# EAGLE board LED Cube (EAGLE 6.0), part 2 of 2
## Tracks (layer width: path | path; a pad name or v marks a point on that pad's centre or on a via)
GND  (via drill 0.4)
  Top 0.406: IC6.1 146.54,70.66 v146.7,70.5 | IC5.1 146.21,53.59 v146.5,53.3 | IC3.1 145.82,35.08 v146.3,34.6 | v146.3,17.6 145.78,18.11 IC2.1 143.08,16.45 140.45,16.45 | C5.1 25.29,76.88 C4.1 25.76,76.86 v26.7,77.8 | C6.1 19.52,72.69 C7.1 | C7.1 19.74,70.77 C9.1 | C7.1 19.74,73.74 C8.1 | C8.1 19.88,74.99 R10.2 17.82,76.88 IC10.18 11.72,76.88 11.4,77.2 11.4,78.7 | C8.1 21.79,74.99 v22,75.2 | X2.5 10.34,92.66 11,92 11,82.6 11.45,82.15 | 11.45,82.15 11.5,82.1 | 11.5,82.1 13.09,82.1 IC10.26 | IC10.25 12.18,81.42 11.5,82.1 | 11.4,78.7 11.4,79.4 | 11.4,79.4 11.4,82.1 11.45,82.15 | IC10.21 11.53,78.83 11.4,78.7 | IC10.7 11.32,79.47 11.4,79.4 | IC11.PC IC11.PB | IC11.PD IC11.PC | IC11.PC 50.73,59.02 v50.9,59.2 50.45,58.75 C22.1 | v43.9,78.1 43.84,78.16 IC14.6 41.46,78.2 35.5,78.2 35.03,78.67 C1.1 | IC14.39 47.3,81.8 v47.2,81.7 | v51,78.3 51.14,78.16 IC14.28 53.16,78.1 60.7,78.1 | IC14.18 v48.1,74.5 | 60.7,78.1 60.9,78.1 62.02,76.98 C2.2 63.1,76.44 U$74.B2 U$74.B | C3.2 60.14,77.54 60.7,78.1 | R27.2 18.99,39.51 v19.3,39.2 | R28.2 27.19,39.51 v27.3,39.4 | R29.2 35.39,39.51 v35.6,39.3 | R30.2 43.49,39.51 v43.7,39.3 | v19.7,52.9 19.59,53.01 R23.2 18.28,50.82 U$70.3 | R24.2 27.29,52.91 v27.4,52.8 | R25.2 v35.89,52.81 v35.9,52.8 | R26.2 43.69,52.71 v43.9,52.5 | C14.2 34.91,21.12 C15.2 35.52,22.48 v36.3,21.7 | R31.1 53.49,11.37 R21.1 53.03,11.33 v52,10.3 | C12.2 26.14,16.24 24.15,14.25 | 24.15,14.25 24.1,14.2 24.1,11.7 23.1,10.7 20.17,10.7 IC12.2 | C10.1 21.86,16.54 24.15,14.25 | C11.2 34.61,8.11 v35,8.5 | 44.3,25.19 IC1.3 51.8,25.2 52.61,24.39 IC1.21 57.64,24.39 C18.2 59.64,24.74 C17.2 60.49,23.91 59.7,24.7 57.8,24.7 57.8,24.5 57.7,24.4 54.3,24.4 v53.6,23.7
  Top 0.406: 44.3,25.19 43.84,25.19 C16.2 | IC1.5 45.9,23.59 44.3,25.19 | C19.2 5.4,31.55 C20.2 3.85,32.7 IC13.GND | R14.1 47.7,67.2 v47.9,67.4 | IC9.10 77.13,84.27 78.5,82.9 C23.1 80.65,83.95 v80.1,84.5 | IC9.1 79.42,96.97 v79.7,96.7 | IC8.10 79.14,65.1 C24.1 80.35,66.15 v79.8,66.7 | IC8.1 79.14,78.83 v79.5,79.2 | IC4.10 76.45,44.85 77.2,44.1 80.25,44.1 C25.1 80.35,45.15 v80,45.5 | IC4.1 78.67,58.27 v79.4,59 | C26.1 78.3,22.7 78.2,22.8 | 76.5,24.5 76.5,25.2 IC7.10 76.55,24.55 76.5,24.5 | IC7.1 78.69,36.69 v79.1,37.1 | 76.5,24.5 78.2,22.8 | 78.2,22.8 78.2,23.6 v78.4,23.8 | C27.1 140.45,16.45 | 140.45,16.45 139,17.9 139,29 139.6,29.6 144.69,29.6 IC2.10 | v142,32.6 C28.1 140.5,32.65 140.5,34.7 138.7,36.5 138.7,45.7 139.5,46.51 IC3.10 | v142.2,50.9 142.1,51 C29.1 140.6,51.05 140.6,53.3 138.8,55.1 138.8,64.3 139.53,65.03 IC5.10 | v142.5,68.4 142.3,68.2 C30.1 140.7,68.25 140.7,81.3 141.49,82.08 IC6.10
  Bottom 0.406: v146.7,70.5 146.5,70.5 | v146.5,53.3 146.1,53.3 | v146.3,34.6 146,34.6 | v146.3,17.6 145.9,17.6 | v26.7,77.8 26.2,77.8 | v22,75.2 21.9,75.2 21.8,75.3 | v50.9,59.2 53.5,59.2 | v43.9,78.1 43.6,78.1 | v47.2,81.7 47.2,82.1 47.3,82.2 | v51,78.3 51.3,78.3 51.4,78.2 | v48.1,74.5 48.1,74 48.2,74 | v19.3,39.2 18.9,39.2 18.8,39.1 | v27.3,39.4 27.1,39.4 26.9,39.2 | v35.6,39.3 35.5,39.3 35.3,39.1 | v43.7,39.3 43.6,39.3 43.3,39 | v19.7,52.9 19.5,52.9 19.4,52.8 | v27.4,52.8 27.2,52.8 27.1,52.7 | v35.9,52.8 35.9,52.7 35.7,52.5 | v43.9,52.5 43.8,52.5 43.7,52.4 | v36.3,21.7 35.7,21.7 | v52,10.3 52,10.8 | v35,8.5 34.6,8.5 | v47.9,67.4 47.9,67 48,66.9 | v80.1,84.5 80.1,84 | v79.7,96.7 79.3,96.7 79.2,96.6 | v79.8,66.7 79.8,66.1 | v79.5,79.2 79.2,79.2 79.1,79.3 | v80,45.5 80,45.2 | v79.4,59 78.6,59 | v79.1,37.1 78.7,37.1 78.6,37.2 | v78.4,23.8 78.4,23.5 | v142,32.6 142,32.2 | v142.2,50.9 142,50.9 | v142.5,68.4 142.1,68.4 | v53.6,23.7 53.6,24
  pour Bottom (isolate 0.4): 0,0 160,0 160,100 0,100
  pour Top (isolate 0.4): 0,0 160,0 160,100 0,100
N$1  (via drill 0.4)
  Top 0.406: U$3.P$3 99.96,32.54 100.8,31.7 104.9,31.7 108.2,28.4 108.2,22.2 108.4,22 108.4,21.1 107.1,19.8 v107.1,19.5
  Bottom 0.406: v107.1,19.5 111.09,19.5 SV1.4
N$2
  Top 0.406: IC14.4 36.94,79.76 32.5,84.2 32.5,86.2 | 32.5,86.2 32.5,93.72 JP3.5 | R1.2 32.5,86.2
N$3
  Top 0.406: IC14.29 62.28,78.96 C2.1
N$4  (via drill 0.4)
  Top 0.406: IC6.2 150.07,71.92 150.5,71.5 v150.5,55 v150.5,36.3 v150.5,19.4 150.5,10.8 149.7,10 106.3,10 104.5,11.8 104.5,14.8 99.3,20 75.7,20 72.4,23.3 72.4,25.3 74,25.3 74.2,25.5 74.2,25.6 74.4,25.8 v74.4,36 v74.4,57.1 v74.4,77.8 74.4,95.4 74.5,95.5 | v142.2,55 144.81,55 IC5.2 | IC2.2 140.81,19.39 v140.8,19.4 | IC7.2 80.58,35.41 v80.6,35.4 | IC4.2 v80.39,56.99 v80.4,57 | IC8.2 80.86,77.56 v80.9,77.6 | 74.5,95.5 74.7,95.7 IC9.2 | IC14.37 48.9,87.1 51.6,89.8 57.5,89.8 57.9,90.2 57.9,92 61.5,95.6 74.4,95.6 74.5,95.5 | IC3.2 142.06,36.34 v142,36.4
  Bottom 0.406: v150.5,55 v142.2,55 | v140.8,19.4 v150.5,19.4 | v80.6,35.4 75,35.4 v74.4,36 | v80.4,57 74.5,57 v74.4,57.1 | v80.9,77.6 74.6,77.6 v74.4,77.8 | v142,36.4 150.4,36.4 v150.5,36.3
N$5  (via drill 0.4)
  Top 0.406: IC6.3 151.1,73.19 151.5,72.8 v151.5,56.2 v151.5,37.6 v151.5,20.6 151.5,10.7 150.1,9.3 105.8,9.3 103.6,11.5 103.6,14.5 99,19.1 75.4,19.1 71.7,22.8 71.7,25.5 72.2,26 73.1,26 73.4,26.3 v73.4,34.8 v73.4,55.9 v73.4,76.6 v73.4,94.5 61.6,94.5 58.8,91.7 58.8,89.4 58.3,88.9 52,88.9 49.7,86.6 IC14.36 | v140.9,56.2 144.88,56.2 IC5.3 | IC2.3 142.16,20.66 v142.1,20.6 | IC7.3 79.25,34.15 v79.3,34.2 | IC4.3 79.12,55.73 v79.2,55.8 | IC8.3 v79.69,76.3 v79.7,76.3 | v81.2,94.5 77.2,94.5 IC9.3 | IC3.3 140.72,37.62 v140.7,37.6
  Bottom 0.406: v151.5,56.2 v140.9,56.2 | v142.1,20.6 v151.5,20.6 | v79.3,34.2 74,34.2 v73.4,34.8 | v79.2,55.8 73.5,55.8 v73.4,55.9 | v79.7,76.3 73.7,76.3 v73.4,76.6 | v73.4,94.5 v81.2,94.5 | v140.7,37.6 v151.5,37.6
N$6  (via drill 0.4)
  Top 0.406: IC6.4 152.13,74.47 152.3,74.3 v152.3,57.4 v152.3,38.9 v152.3,21.9 152.3,10.3 150.7,8.7 146.3,8.6 105.4,8.6 102.8,11.2 102.8,14.2 98.6,18.4 75,18.4 71,22.4 71,25.9 71.8,26.7 72.2,26.7 72.4,26.9 v72.4,32.6 v72.4,54.3 v72.4,75.1 v72.4,93.2 61.7,93.2 59.7,91.2 59.7,88.8 58.9,88 52.3,88 50.5,86.2 IC14.35 | v142.2,57.4 IC5.4 | IC3.4 141.91,38.88 v141.9,38.9 | IC7.4 80.47,32.88 v80.5,32.9 | IC4.4 80.34,54.45 v80.4,54.4 | IC8.4 80.78,75.03 v80.8,75 | v79.8,93.2 77.17,93.2 IC9.4 | IC2.4 140.88,21.93 v140.8,22
  Bottom 0.406: v152.3,57.4 v142.2,57.4 | v141.9,38.9 v152.3,38.9 | 152.1,21.9 152.2,22 | 152.28,21.93 v152.3,21.9 152.2,22 | v80.5,32.9 72.7,32.9 v72.4,32.6 | v80.4,54.4 72.5,54.4 v72.4,54.3 | v80.8,75 72.5,75 v72.4,75.1 | v72.4,93.2 v79.8,93.2 | v140.8,22 152.2,22
N$7
  Top 0.406: IC14.7 32.63,77.36 Q1.2 25.41,79.94 C5.2
N$8
  Top 0.406: IC14.8 31.49,76.56 Q1.1 25.35,75.12 C4.2
N$9  (via drill 0.4)
  Top 0.406: IC6.5 152.97,75.73 153.2,75.5 153.2,58.8 v153.1,58.7 | v140.9,58.7 144.92,58.7 IC5.5 | IC3.5 140.84,40.16 v140.8,40.2 | v153.1,58.7 v153.1,40.2 v153.1,23.2 | IC2.5 v142.1,23.2 | v153.1,58.7 153.1,9.9 151.2,8 104.9,8 102,10.9 102,13.9 98.2,17.7 74.6,17.7 70.3,22 70.3,26.1 71.1,26.9 v71.1,32.1 v71.1,53.4 v71.1,73.8 71.1,91.8 | IC7.5 79.11,31.61 v79.2,31.7 | IC4.5 78.89,53.19 v79,53.3 | IC8.5 79.56,73.75 v79.6,73.8 | 71.1,91.8 v71.2,91.9 | v81,91.9 IC9.5 | 71.1,91.8 62.3,91.8 60.7,90.2 60.7,88.2 59.6,87.1 52.8,87.1 51.3,85.6 IC14.34
  Bottom 0.406: v140.8,40.2 v153.1,40.2 | v142.1,23.2 v153.1,23.2 | v79.2,31.7 71.5,31.7 v71.1,32.1 | v79,53.3 71.2,53.3 v71.1,53.4 | v79.6,73.8 v71.1,73.8 | v71.2,91.9 v81,91.9 | v153.1,58.7 144.97,58.7 IC5.5 140.93,58.67 v140.9,58.7 v153.1,58.7
N$10  (via drill 0.4)
  Top 0.406: IC6.6 153.79,77 154,76.8 v154,60 v154,41.6 v154,24.6 154,9.5 151.7,7.2 104.5,7.2 101.1,10.6 101.1,13.5 97.8,16.8 74.2,16.8 69.4,21.6 69.4,26.8 69.5,26.9 69.6,26.9 69.7,27 v69.7,30.4 v69.7,52.2 v69.7,72.9 v69.7,90.6 69.6,90.7 62.6,90.7 61.8,89.9 61.8,83 60.96,82.16 IC14.33 | v142.2,60 144.89,60 IC5.6 | IC3.6 142.07,41.42 v142,41.5 | IC2.6 140.94,24.46 v140.8,24.6 | IC7.6 80.33,30.34 v80.4,30.4 | IC4.6 80.28,51.91 v80.3,51.9 | IC8.6 80.78,72.48 v80.8,72.5 | v79.7,90.6 77.16,90.6 IC9.6
  Bottom 0.406: v154,60 v142.2,60 | v142,41.5 154,41.5 v154,41.6 | v140.8,24.6 v154,24.6 | v80.4,30.4 v69.7,30.4 | v80.3,51.9 70,51.9 v69.7,52.2 | v80.8,72.5 70.1,72.5 v69.7,72.9 | v69.7,90.6 v79.7,90.6
N$11  (via drill 0.4)
  Top 0.406: IC6.7 154.62,78.28 154.8,78.1 v154.8,61.2 v154.8,42.7 v154.8,25.8 154.8,9.1 152.2,6.5 152.2,6.4 104.1,6.4 100.2,10.3 100.2,13.2 97.4,16 73.7,16 68.5,21.2 68.5,26.9 68.2,27.2 v68.2,28.9 v68.2,51 v68.2,71.2 v68.2,89.4 63.4,89.4 62.6,88.6 62.6,82.5 61.46,81.36 IC14.32 | v140.9,61.2 144.93,61.2 IC5.7 | IC2.7 142.16,25.73 v142.1,25.8 | IC7.7 78.97,29.07 v79,29.1 | IC4.7 78.94,50.65 v79,50.7 | IC8.7 79.39,71.22 v79.4,71.2 | v81.1,89.4 77.18,89.4 IC9.7 | IC3.7 v140.71,42.7 v140.7,42.7
  Bottom 0.406: v154.8,61.2 v140.9,61.2 | v142.1,25.8 v154.8,25.8 | v79,29.1 68.4,29.1 v68.2,28.9 | v79,50.7 68.5,50.7 v68.2,51 | v79.4,71.2 v68.2,71.2 | v68.2,89.4 v81.1,89.4 | v154.79,42.7 v154.8,42.7 v140.7,42.7
N$12  (via drill 0.4)
  Top 0.406: IC6.8 155.35,79.55 155.6,79.3 v155.6,62.5 v155.6,44.1 v155.6,26.9 155.6,8.5 152.7,5.6 103.6,5.6 99.1,10.1 99.1,13 96.9,15.2 73.2,15.2 67.4,21 67.4,26.5 66.6,27.3 v66.6,27.8 v66.6,49.3 v66.6,69.7 v66.6,88.2 64.3,88.2 63.5,87.4 63.5,82.1 61.96,80.56 IC14.31 | v142.2,62.5 144.93,62.5 IC5.8 | IC3.8 142.13,43.97 v142.1,44 | IC7.8 v80.39,27.8 v80.4,27.8 | IC4.8 80.28,49.38 v80.3,49.4 | IC8.8 80.56,69.94 v80.6,69.9 | v79.8,88.1 77.15,88.1 IC9.8 | IC2.8 v140.5,27
  Bottom 0.406: v155.6,62.5 v142.2,62.5 | v142.1,44 155.5,44 v155.6,44.1 | v80.4,27.8 v66.6,27.8 | v80.6,69.9 66.8,69.9 v66.6,69.7 | v66.6,88.2 79.7,88.2 v79.8,88.1 | v140.5,27 155.6,27 v155.6,26.9 | v80.3,49.4 66.6,49.4 v66.6,49.3
N$13  (via drill 0.4)
  Top 0.406: IC6.9 155.69,80.81 156.4,80.1 v156.4,63.7 | v140.9,63.8 144.9,63.8 IC5.9 | IC3.9 140.76,45.23 v140.7,45.3 | v156.4,63.7 v156.4,45.5 v156.4,28.4 | IC2.9 142.03,28.27 v142,28.3 | v156.4,63.7 156.4,8 153.3,4.9 103.3,4.9 98.4,9.8 98.4,12.6 96.5,14.5 72.7,14.5 66.5,20.7 66.5,25.6 64.9,27.2 v64.9,27.3 v64.9,48.1 v64.9,68.8 64.9,79.8 | IC7.9 78.83,26.52 v78.9,26.6 | IC4.9 v78.89,48.1 v78.9,48.1 | IC8.9 79.28,68.67 v79.3,68.7 | 64.9,79.8 64.9,86.7 v65,86.8 | v81,86.9 77.22,86.9 IC9.9 | IC14.30 64.86,79.76 64.9,79.8
  Bottom 0.406: v140.7,45.3 156.2,45.3 v156.4,45.5 | v142,28.3 156.3,28.3 v156.4,28.4 | v78.9,26.6 65.6,26.6 v64.9,27.3 | v78.9,48.1 v64.9,48.1 | v79.3,68.7 65,68.7 v64.9,68.8 | v65,86.8 80.9,86.8 v81,86.9 | v156.4,63.7 141,63.7 v140.9,63.8 156.3,63.8 v156.4,63.7
N$14  (via drill 0.4)
  Top 0.406: IC9.11 87.19,84.99 v86.3,84.1 | v59.1,85.1 54.3,85.1 v52.7,83.5 | v44.9,87.7 45.3,87.7 45.7,87.3 IC14.41
  Bottom 0.406: v86.3,84.1 86.3,83.6 85.4,82.7 61.5,82.7 v59.1,85.1 | v52.7,83.5 49.1,83.5 v44.9,87.7
N$15  (via drill 0.4)
  Top 0.406: IC8.11 86.89,65.59 v86,64.7 | v44.9,81.7 IC14.42 | v57.3,59.6 61.7,59.6 v62.3,59
  Bottom 0.406: v44.9,81.7 45.1,81.5 45.1,66.4 46.8,64.7 55.3,64.7 57.5,62.5 57.5,59.8 v57.3,59.6 | v62.3,59 63.1,59 68.65,64.55 68.8,64.7 v86,64.7
N$16  (via drill 0.4)
  Top 0.406: IC6.11 134.99,83.11 v132.8,85.3 | IC14.21 50.5,74.2 v49.3,75.4 | v46.2,77.3 46.2,77.2 v43.4,74.4 | v71,11.2 82.5,11.2 v84.8,8.9
  Bottom 0.406: v132.8,85.3 130.6,85.3 125.3,80 125.3,11.7 122.4,8.8 97,8.8 96.9,8.9 v84.8,8.9 | v49.3,75.4 49.3,77.6 48.4,78.5 47.4,78.5 v46.2,77.3 | v43.4,74.4 43.4,65.5 44.1,64.8 44.1,57.5 46.5,55.1 48.1,55.1 53.3,49.9 53.3,47.7 59.2,41.8 59.2,24.3 61.5,22 64.9,22 70.6,16.3 70.6,11.6 v71,11.2
N$17  (via drill 0.4)
  Top 0.406: IC5.11 134.18,65.03 v132.6,66.6 | IC14.22 53.16,72.36 v53.6,72.8 | v54,83.1 v58.8,83.1 | v63.2,48.5 63.2,26.8 v64.6,25.4
  Bottom 0.406: v132.6,66.6 127.5,66.6 126.5,65.6 126.5,11.3 122.7,7.5 83.7,7.5 65.8,25.4 v64.6,25.4 | v53.6,72.8 53.6,82.7 v54,83.1 | v58.8,83.1 58.8,82.2 63.4,77.6 63.4,66.4 61.4,64.4 61.4,58.5 63.4,56.5 63.4,48.7 v63.2,48.5
N$18  (via drill 0.4)
  Top 0.406: IC4.11 86.51,44.71 v85.4,43.6 | v60.3,62.8 60.3,66.7 v60.4,66.8 | v57.4,74.1 53.16,74.1 IC14.23
  Bottom 0.406: v85.4,43.6 65.3,43.6 60.3,48.6 v60.3,62.8 | v60.4,66.8 60.4,71.1 v57.4,74.1
N$19  (via drill 0.4)
  Top 0.406: IC3.11 133.59,46.51 v132.5,47.6 | IC14.24 50.94,74.96 v50.6,75.3 | v46.4,79.9 v43,79.9 | v74,6.3 v80.5,6.3
  Bottom 0.406: v132.5,47.6 128.7,47.6 127.9,46.8 127.9,11 123.2,6.3 v80.5,6.3 | v50.6,75.3 50.6,77.4 48.2,79.8 46.5,79.8 v46.4,79.9 | v43,79.9 43,79.1 41.6,77.6 41.6,66.2 43.3,64.5 43.3,57.1 46,54.4 47.7,54.4 52.5,49.6 52.5,47.3 58.4,41.4 58.4,23.9 61.2,21.1 64.6,21.1 69.8,15.9 69.8,10.5 v74,6.3
N$20  (via drill 0.4)
  Top 0.406: IC2.11 134.16,29.55 v133.1,30.6 | v53.9,62.7 53.8,62.7 53.3,63.2 53.3,66.7 v53.1,66.9 | v48.3,76.6 50.4,76.6 51.2,75.8 53.06,75.8 IC14.25
  Bottom 0.406: v133.1,30.6 130.7,30.6 129.3,29.2 129.3,10.6 123.8,5.1 79.1,5.1 71.5,12.7 71.5,16.6 60.2,27.9 60.2,42.1 54.6,47.7 54.6,62 v53.9,62.7 | v53.1,66.9 53.1,66.6 52.1,65.6 47.3,65.6 46,66.9 46,74.3 v48.3,76.6
N$21  (via drill 0.4)
  Top 0.406: IC7.11 86.61,24.39 v87.8,23.2 | v58.5,67.3 58.7,67.3 61.2,69.8 61.2,74.4 v60.5,75.1 | v56.9,76.4 56.8,76.4 56.6,76.6 53.14,76.6 IC14.26
  Bottom 0.406: v87.8,23.2 87.8,37.1 85.2,39.7 65.7,39.7 58.5,46.9 v58.5,67.3 | v60.5,75.1 58.2,75.1 v56.9,76.4
N$22
  Top 0.406: R23.1 16.58,56.94 U$66.1 16.95,56.61 R2.2
N$23
  Top 0.406: IC14.16 46.5,70 42,65.5 22.2,65.5 20.2,63.5 20.2,58.35 R2.1
N$24  (via drill 0.4)
  Top 0.406: IC14.15 45.7,70.3 41.7,66.3 v28.4,66.3 | v28.4,64.2 28.4,57.88 R3.1
  Bottom 0.406: v28.4,66.3 v28.4,64.2
N$25  (via drill 0.4)
  Top 0.406: IC14.14 44.9,70.6 41.4,67.1 37.8,67.1 v37.6,67.3 | v36.6,62.6 36.6,57.89 R4.1
  Bottom 0.406: v37.6,67.3 37.6,63.6 v36.6,62.6
N$26  (via drill 0.4)
  Top 0.406: v38.2,62.6 38.2,52.7 39.8,51.1 46.7,51.1 47.4,51.8 47.4,52.8 R5.1 | IC14.13 44.1,70.7 41.3,67.9 v39.2,67.9
  Bottom 0.406: v39.2,67.9 39.2,63.6 v38.2,62.6
N$27  (via drill 0.4)
  Top 0.406: R6.1 19.86,51.06 21.5,52.7 21.5,62.2 | 21.5,62.2 21.5,62.5 v21.3,62.7 21.3,62.4 21.5,62.2 | IC14.12 43.3,71.6 41.7,70 v39.4,70
  Bottom 0.406: v39.4,70 24.9,70 21.3,66.4 v21.3,62.7
N$28  (via drill 0.4)
  Top 0.406: R7.1 28.06,49.96 29.9,51.8 v29.9,63 | v30.4,68.8 34,68.8 36.2,71 36.2,72.2 v35.9,72.5 | v39.1,72.8 39.1,73.5 39.7,74.1 41.44,74.1 IC14.11
  Bottom 0.406: v29.9,63 29.9,68.3 v30.4,68.8 | v35.9,72.5 38.8,72.5 v39.1,72.8
N$29  (via drill 0.4)
  Top 0.406: R8.1 37.13,44.87 37.6,44.4 37.6,38.2 36.7,37.3 14,37.3 11.8,39.5 11.8,62.2 v12.4,62.8 | v41.9,86.2 42.9,86.2 43.3,85.8 IC14.44
  Bottom 0.406: v12.4,62.8 12.4,63.7 17,68.3 19.2,68.3 24.3,73.4 24.3,76.5 22.5,78.3 22.5,84.9 24.2,86.6 41.5,86.6 v41.9,86.2
N$30  (via drill 0.4)
  Top 0.406: IC14.43 44.1,86.3 v42.9,87.5 | v11,63.6 11,39.2 13.6,36.6 44.2,36.6 46.4,38.8 46.4,43.7 45.6,44.5 44.84,44.5 R9.1
  Bottom 0.406: v42.9,87.5 23.8,87.5 21.7,85.4 21.7,77.8 23.4,76.1 23.4,73.8 18.8,69.2 16.6,69.2 v11,63.6
N$31
  Top 0.406: R24.1 24.6,56.76 U$67.1 25.44,56.12 R3.2
N$32
  Top 0.406: R25.1 33.12,56.88 U$68.1 34.03,56.13 R4.2
N$33
  Top 0.406: R26.1 41.14,56.7 U$69.1 45.12,52.84 R5.2
N$34
  Top 0.406: R27.1 16.36,43.82 U$70.1 16.61,43.65 R6.2
N$35
  Top 0.406: R28.1 24.28,43.64 U$71.1 24.9,43.26 R7.2
N$36
  Top 0.406: R29.1 32.7,43.46 U$72.1 33.19,43.17 R8.2
N$37
  Top 0.406: R30.1 40.72,43.48 U$73.1 41.38,42.98 R9.2
N$38
  Bottom 0.406: JP1.1 3.32,60.72 3.6,61 10.7,61 12.2,59.5 U$66.2
N$39
  Bottom 0.406: JP1.2 11.7,58.8 12.2,58.3 20.9,58.3 22,59.4 U$67.2
N$42
  Bottom 0.406: JP1.5 3.32,53.58 4.5,52.4 8.7,52.4 12.1,49 12.1,47.2 12.9,46.4 U$70.2
N$43
  Bottom 0.406: JP1.6 9.08,53.72 10.3,52.5 18.3,52.5 20,50.8 20,47.2 20.9,46.3 U$71.2
N$44
  Bottom 0.406: JP1.7 3.32,51.08 4.6,49.8 8.3,49.8 10.3,47.8 10.3,43.9 13.7,40.5 25.9,40.5 28.2,42.8 28.2,44.9 29.4,46.1 U$72.2
N$45
  Bottom 0.406: JP1.8 8.42,51.18 11.2,48.4 11.2,46.1 12.2,45.1 26.8,45.1 29.2,47.5 36.5,47.5 37.9,46.1 U$73.2
N$46
  Top 0.406: X2.1 15.54,95.86 18,93.4 18,82.72 R11.2
N$47
  Top 0.406: IC14.3 37.44,80.56 35.1,82.9 35.1,93.78 JP3.7
N$48
  Top 0.406: IC14.2 38.34,81.36 37.7,82 37.7,93.8 JP3.9
N$49  (via drill 0.4)
  Top 0.406: v39.2,91.2 39.2,82.8 39.8,82.2 41.46,82.2 IC14.1
  Bottom 0.406: JP3.1 27.52,92.28 28.2,91.6 38.8,91.6 v39.2,91.2
N$50  (via drill 0.4)
  Top 0.406: IC14.10 38.46,74.96 38.2,74.7 38.2,69.5 35.9,67.2 4.9,67.2 v2.5,69.6 | v2.9,80.8 5.84,80.8 IC10.5
  Bottom 0.406: v2.5,69.6 2.5,80.4 v2.9,80.8
N$51
  Top 0.406: IC10.1 2.48,83.38 1.9,82.8 1.9,72 5.9,68 35.2,68 37.2,70 37.2,75.1 37.86,75.76 IC14.9
N$52
  Top 0.406: R11.1 18.04,78.79 R10.1 17.85,78.6 16.9,78.6 15.82,77.53 IC10.19
N$53
  Top 0.406: IC14.20 49.7,70.3 53,70.3 | IC1.27 52.65,42.95 52.7,43 52.7,53.8 53.9,55 53.9,59.1 52,61 IC11.PE 51.99,69.3 53,70.3 | R13.1 54.81,71.61 53.5,70.3 53,70.3
N$54  (via drill 0.4)
  Top 0.406: X2.3 12.24,94.26 v13,93.5 | v12.5,72.9 12.5,74.31 IC10.15
  Bottom 0.406: v13,93.5 13,73.4 v12.5,72.9
N$55
  Top 0.406: C6.2 17.99,74.61 16.4,76.2 13.14,76.2 IC10.17
N$56  (via drill 0.4)
  Top 0.406: X2.2 14.04,95.06 v15,94.1 | v14.5,73.3 14.5,75.1 14,75.6 13.14,75.6 IC10.16
  Bottom 0.406: v15,94.1 15,73.8 v14.5,73.3
N$57  (via drill 0.4)
  Top 0.406: IC14.19 v48.9,69.1 50.2,69.1 50.73,68.58 IC11.PF 50.7,62.23 50.7,60.6 51,60.3 51.6,60.3 53.1,58.8 53.1,55.4 51.9,54.2 51.9,42.6 51.85,42.55 IC1.28 | R12.1 54.61,69.51 v54.2,69.1
  Bottom 0.406: v54.2,69.1 v48.9,69.1
N$58
  Top 0.406: IC11.PG 49.45,65.66 R14.2
N$59
  Top 0.406: IC12.8 27.84,13.33 C12.1 27.84,19.23 R15.2
N$60
  Top 0.406: IC12.6 31.82,8.18 C11.1
N$61
  Top 0.406: C13.2
  Top 0.813: IC12.5 C13.2
N$62
  Top 0.813: C13.1 25.88,1.71 R16.2 17.16,1.73 R17.2
N$63
  Top 0.813: R16.1 9.58,1.71 U$1.RIGHT
N$64
  Top 0.813: R17.1 13.1,4.21 U$1.LEFT
N$65  (via drill 0.4)
  Top 0.406: IC1.23 54.69,25.99 v54.05,25.35
  Bottom 0.406: IC12.3 22.68,8.18 23.6,9.1 23.6,30 26.9,33.3 53.7,33.3 55.4,35 56.7,35 57.5,34.2 57.5,32.6 54.4,29.5 54.4,25.7 v54.05,25.35 54,25.3
N$66  (via drill 0.4)
  Top 0.406: JP6.5 57.18,5.98 | 57.18,5.98 55.9,4.7 47.5,4.7 46.7,3.9 45.05,3.9 R19.1 | 57.18,5.98 57.18,16.32 56.7,16.8 56.7,19.5 v57.4,20.2 | v51.1,26.4 51.1,28.23 IC1.29
  Bottom 0.406: v57.4,20.2 55.4,20.2 51.1,24.5 v51.1,26.4
N$67  (via drill 0.4)
  Top 0.406: v55.9,33.2 54.4,31.7 54.4,28.43 IC1.25
  Bottom 0.406: IC12.4 23.84,5.64 25,6.8 25,29.3 27.5,31.8 54.5,31.8 v55.9,33.2
N$68  (via drill 0.4)
  Top 0.406: IC1.26 53.45,26.55 v53,26.1
  Bottom 0.406: v53,26.1 53,30.1 52.3,30.8 33.4,30.8 31.4,28.8 31.4,12.4 29.7,10.7 27.79,10.7 IC12.7
N$69  (via drill 0.4)
  Top 0.406: IC14.40 v46.5,89.3 R20.2 | U$74.A U$74.A2 v55.6,68.2
  Bottom 0.406: v55.6,68.2 55.6,83 49.3,89.3 v46.5,89.3
N$70
  Top 0.406: IC1.8 41.05,21.19 Q10.1 35.1,19.19 C14.1
N$71
  Top 0.406: IC1.7 41.07,21.99 Q10.2 38.88,24.18 C15.1
N$74
  Top 0.406: X1.2 5.02,29.47 C20.1 | IC13.IN 3.44,30.16 3.9,29.7 5.15,29.7 C20.1 | C21.+ 6.89,27.96 C20.1
N$75
  Top 0.406: IC1.14 52.55,17.77 LED65.A
N$76
  Top 0.406: R21.2 53.53,15.29 LED65.C
N$77
  Top 0.406: R18.S 62.13,25.37 60.8,26.7 55.83,26.7 IC1.24
N$78
  Top 0.406: IC1.20 57.44,23.59 C18.1
N$79
  Top 0.406: JP6.9 52.25,9.05 53.2,10 54.6,10 55.2,10.6 55.2,18.75 IC1.16
N$80  (via drill 0.4)
  Top 0.406: JP6.1 62.41,7.59 57.8,12.2 v57.8,18 | v53.5,18.3 53.5,19.65 IC1.15
  Bottom 0.406: v57.8,18 53.8,18 v53.5,18.3
N$81
  Top 0.406: JP6.7 54.79,8.89 56,10.1 56,20.93 IC1.17
N$82
  Top 0.406: R31.2 51.33,15.33 LED1.C
N$83
  Top 0.406: IC1.13 51.75,17.25 LED1.A
N$84
  Top 0.406: IC13.OUT 2.84,35.24 4.1,36.5 5.35,36.5 C19.1 5.43,36.58 JP2.1
N$98  (via drill 0.4)
  Top 0.406: U$5.P$3 100.56,36.84 101.5,35.9 105.7,35.9 109.7,31.9 109.7,18.9 v108.3,17.5
  Bottom 0.406: v108.3,17.5 109.7,17.5 111.3,15.9 112.15,15.9 SV1.2
N$99  (via drill 0.4)
  Top 0.406: U$6.P$3 105.86,34.54 109,31.4 109,19.9 v107.6,18.5
  Bottom 0.406: v107.6,18.5 110.1,18.5 111.9,16.7 113.73,16.7 SV1.3
N$100  (via drill 0.4)
  Top 0.406: U$4.P$3 104.86,30.44 107.2,28.1 107.2,21.8 v107.5,21.5
  Bottom 0.406: v107.5,21.5 111.7,21.5 112,21.8 113.87,21.8 SV1.5
N$101
  Top 0.406: R44.2 96.67,27.76 U$7.P$1
N$102  (via drill 0.4)
  Top 0.406: U$7.P$3 100.86,28.54 102.1,27.3 105.6,27.3 106.2,26.7 106.2,20.7 v106.3,20.6
  Bottom 0.406: v106.3,20.6 111.73,20.6 SV1.6
N$103
  Top 0.406: R42.2 96.58,36.11 U$5.P$1
N$104  (via drill 0.4)
  Top 0.406: U$9.P$3 100.56,24.24 v102.4,22.4
  Bottom 0.406: v102.4,22.4 111.81,22.4 SV1.8
N$105
  Top 0.406: U$17.P$3 119.95,29.95 118.5,31.4 118.5,32.9 116.8,34.6 113.85,34.6 SV1.16
N$106
  Top 0.406: R63.2 102.02,59.76 U$26.P$1
N$107
  Top 0.406: R64.2 96.54,53.36 U$27.P$1
N$108
  Top 0.406: R65.2 102.26,51.26 U$28.P$1
N$109
  Top 0.406: U$11.P$3 119.65,21.45 118.3,22.8 118.3,24.5 117,25.8 117,28 115.6,29.4 113.73,29.4 SV1.12
N$110
  Top 0.406: U$13.P$3 119.25,17.35 118.2,18.4 118.2,21 116.8,22.4 116.8,23.8 116.3,24.3 113.91,24.3 SV1.10
N$111  (via drill 0.4)
  Top 0.406: U$10.P$3 119.85,15.25 117.1,18 117.1,20.5 v117,20.6
  Bottom 0.406: v117,20.6 117,23.75 SV1.9
N$112
  Top 0.406: R54.2 122.16,30.64 U$17.P$1
N$113
  Top 0.406: IC4.19 89.25,56.99 R63.1
N$114
  Top 0.406: IC4.16 91.86,53.19 R64.1
N$115
  Top 0.406: R66.2 96.43,57.61 U$29.P$1
N$116
  Top 0.406: IC4.18 90.16,55.73 R66.1
N$117
  Top 0.406: R67.2 102.05,55.51 U$30.P$1
N$118
  Top 0.406: IC4.17 91,54.45 R67.1
N$119
  Top 0.406: IC4.15 91.41,51.91 R65.1
N$120
  Top 0.406: R68.2 96.57,49.11 U$31.P$1
N$121
  Top 0.406: R71.2 126.2,51.59 U$34.P$1
N$122
  Top 0.406: R72.2 122.68,57.89 U$35.P$1
N$123
  Top 0.406: R73.2 126.26,59.99 U$36.P$1
N$124
  Top 0.406: IC5.19 133.34,54.87 R71.1
N$125
  Top 0.406: IC5.16 130.93,58.67 R72.1
N$126
  Top 0.406: R74.2 122.54,53.69 U$37.P$1
N$127
  Top 0.406: IC5.18 132.44,56.13 R74.1
N$128
  Top 0.406: R75.2 126.22,55.79 U$38.P$1
N$129
  Top 0.406: IC7.19 88.78,35.41 R39.1
N$130
  Top 0.406: U$64.P$3 107.87,86.67 108.8,87.6 108.8,93.9 110.5,95.6 113.73,95.6 SV1.63
N$131  (via drill 0.4)
  Top 0.406: U$60.P$3 105.37,90.57 v105.4,90.6
  Bottom 0.406: v105.4,90.6 107.2,90.6 109.6,93 113.79,93 SV1.61
N$132
  Top 0.406: IC7.16 91.3,31.61 R40.1
N$133
  Top 0.406: IC2.19 133.44,19.39 130,15.94 R47.1
N$134  (via drill 0.4)
  Top 0.406: U$63.P$3 100.53,88.47 101.2,87.8 105.1,87.8 v105.4,88.1
  Bottom 0.406: v105.4,88.1 106.1,88.1 109.7,91.8 112.45,91.8 SV1.62
N$135
  Top 0.406: IC2.16 130.94,23.2 R48.1
N$136
  Top 0.406: U$61.P$3 100.53,96.67 101.2,96 104.3,96 105.7,97.4 115.7,97.4 117,96.1 117,89.4 115.5,87.9 113.81,87.9 SV1.58
N$137
  Top 0.406: R95.2 100.9,98.16 U$58.P$1
N$138
  Top 0.406: U$56.P$3 108.27,68.27 109.1,69.1 109.1,82.9 111.6,85.3 113.87,85.3 SV1.55
N$139
  Top 0.406: R96.2 97.22,91.76 U$59.P$1
N$140
  Top 0.406: R97.2 101.04,89.66 U$60.P$1
N$141
  Top 0.406: IC9.19 90.53,95.7 R95.1
N$142  (via drill 0.4)
  Top 0.406: U$55.P$3 100.23,70.37 101.2,69.4 104.5,69.4 v104.6,69.5
  Bottom 0.406: v104.6,69.5 105.6,69.5 107,70.9 107,76.01 SV1.54
N$143
  Top 0.406: IC9.16 92.77,91.89 R96.1
N$144  (via drill 0.4)
  Top 0.406: v101,77.3 101,78.2 100.1,79.1 98.52,79.1 U$53.P$3
  Bottom 0.406: SV1.50 110.77,76.47 109.8,75.5 109.8,68.7 108.4,67.3 104,67.3 102.7,68.6 102.7,75.6 v101,77.3
N$145
  Top 0.406: R87.2 101.02,80.11 U$50.P$1
N$146
  Top 0.406: R88.2 96.69,73.76 U$51.P$1
N$147
  Top 0.406: R89.2 101.21,71.66 U$52.P$1
N$148
  Top 0.406: R88.1 IC8.16
N$149
  Top 0.406: R87.1 89.61,77.56 IC8.19
N$150
  Top 0.406: R90.2 96.53,77.96 U$53.P$1
N$151
  Top 0.406: R90.1 90.52,76.3 IC8.18
N$152
  Top 0.406: R91.2 101.22,75.86 U$54.P$1
N$153
  Top 0.406: R79.2 126.04,69.59 U$42.P$1
N$154
  Top 0.406: R80.2 122.22,75.89 U$43.P$1
N$155
  Top 0.406: R81.2 126.1,77.99 U$44.P$1
N$156
  Top 0.406: IC6.19 132.44,71.92 R79.1
N$157
  Top 0.406: IC6.16 130.24,75.73 R80.1
N$158
  Top 0.406: R82.2 126.19,71.69 126,71.5 122.47,71.5 U$45.P$1
N$159
  Top 0.406: IC6.18 131.65,73.19 R82.1
N$160
  Top 0.406: R83.2 125.56,73.79 U$46.P$1
N$161
  Top 0.406: R40.2 96.54,31.91 U$3.P$1
N$162
  Top 0.406: R39.2 102.02,38.21 U$2.P$1
N$163
  Top 0.406: IC7.15 91.09,30.34 R41.1
N$164
  Top 0.406: U$2.P$3 105.06,38.74 110.5,33.3 110.5,15.5 111.7,14.3 113.87,14.3 SV1.1
N$165
  Top 0.406: U$4.P$1 101.86,28.84 101.5,29.2 99.2,29.2 98.6,29.8 R41.2
N$166  (via drill 0.4)
  Top 0.406: U$8.P$3 104.44,26.14 v104.8,26.5
  Bottom 0.406: v104.8,26.5 105.3,26.5 107.4,24.4 113.81,24.4 SV1.7
N$167
  Top 0.406: IC3.19 133.34,36.34 R55.1
N$168
  Top 0.406: IC3.16 130.94,40.16 R56.1
N$169
  Top 0.406: U$10.P$1 126,15.84 R47.2
N$170
  Top 0.406: IC7.14 90.33,29.07 R44.1
N$171
  Top 0.406: R45.2 101.99,25.66 U$8.P$1
N$172
  Top 0.406: IC7.18 89.58,34.15 R42.1
N$173
  Top 0.406: R43.2 102,34.01 U$6.P$1
N$174
  Top 0.406: R48.2 121.98,22.14 U$11.P$1
N$175
  Top 0.406: IC7.17 90.42,32.88 R43.1
N$176
  Top 0.406: IC7.13 89.42,27.8 R45.1
N$177
  Top 0.406: R46.2 96.61,23.56 U$9.P$1
N$178
  Top 0.406: R49.2 125.86,24.24 U$12.P$1
N$179
  Top 0.406: IC7.12 88.72,26.52 R46.1
N$180
  Top 0.406: U$18.P$3 122.35,32.35 121.4,33.3 119.4,33.3 116.9,35.8 115.11,35.8 SV1.17
N$181  (via drill 0.4)
  Top 0.406: U$26.P$3 104.95,60.35 105.5,59.8 105.5,57.3 108.7,54.1 108.7,47.9 v108.5,47.7
  Bottom 0.406: v108.5,47.7 111.4,47.7 111.9,47.2 113.87,47.2 SV1.25
N$182
  Top 0.406: IC4.14 90.55,50.65 R68.1
N$183
  Top 0.406: U$12.P$3 122.95,23.45 121.9,24.5 119.7,24.5 117.7,26.5 117.7,28.2 116.4,29.5 116.4,30.5 116.2,30.7 115.13,30.7 SV1.13
N$184
  Top 0.406: R50.2 122.04,17.94 U$13.P$1
N$185
  Top 0.406: IC2.18 132.66,20.66 R50.1
N$186
  Top 0.406: R51.2 125.92,20.04 U$14.P$1
N$187
  Top 0.406: IC2.17 131.81,21.93 R51.1
N$188
  Top 0.406: U$14.P$3 122.95,19.35 121.8,20.5 119.6,20.5 117.7,22.4 117.7,24.1 116.4,25.4 116.4,26.89 SV1.11
N$189
  Top 0.406: IC2.15 130.09,24.46 R49.1
N$190
  Top 0.406: R69.2 102.26,47.01 U$32.P$1
N$191
  Top 0.406: IC4.13 89.73,49.38 R69.1
N$192
  Top 0.406: R52.2 122.1,26.34 121.39,27.05 U$15.P$1
N$193
  Top 0.406: IC2.14 130.41,25.73 R52.1
N$194
  Top 0.406: U$15.P$3 119.85,25.65 118.4,27.1 118.4,28.5 117.1,29.8 117.1,31.5 116.7,31.9 116.6,31.9 116.5,32 113.79,32 SV1.14
N$195
  Top 0.406: R53.2 125.88,28.44 U$16.P$1
N$196
  Top 0.406: IC2.13 131.31,27 R53.1
N$197
  Top 0.406: U$16.P$3 122.85,27.65 121.8,28.7 119.3,28.7 117.8,30.2 117.8,32.2 116.7,33.3 SV1.15
N$198
  Top 0.406: IC4.12 88.83,48.1 R70.1
N$199
  Top 0.406: U$33.P$3 100.04,45.56 101.4,44.2 107.4,44.2 110.5,47.3 110.5,51.57 SV1.32
N$200
  Top 0.406: IC2.12 132.22,28.27 R54.1
N$201
  Top 0.406: R55.2 126.14,32.84 U$18.P$1
N$202
  Top 0.406: R56.2 122.52,39.14 U$19.P$1
N$203
  Top 0.406: R57.2 126.1,41.24 U$20.P$1
N$204
  Top 0.406: U$34.P$3 120.29,50.94 SV1.33
N$205
  Top 0.406: U$42.P$3 118.34,68.74 115.9,66.3 SV1.41
N$206
  Top 0.406: R58.2 122.48,34.94 U$21.P$1
N$207
  Top 0.406: IC3.18 132.56,37.62 R58.1
N$208
  Top 0.406: R59.2 126.06,37.04 U$22.P$1
N$209
  Top 0.406: IC3.17 131.71,38.88 R59.1
N$210
  Top 0.406: IC3.15 130.09,41.42 R57.1
N$211
  Top 0.406: R60.2 122.54,43.34 U$23.P$1
N$212
  Top 0.406: IC3.14 130.59,42.7 R60.1
N$213
  Top 0.406: R61.2 126.02,45.44 U$24.P$1
N$214
  Top 0.406: IC3.13 131.4,43.97 R61.1
N$215
  Top 0.406: IC3.12 132.21,45.23 R62.1
N$216
  Top 0.406: U$25.P$3 118.75,46.95 116.5,44.7 113.79,44.7 SV1.24
N$217
  Top 0.406: U$24.P$3 123.05,44.75 122.2,45.6 118.5,45.6 116.4,43.5 115.13,43.5 SV1.23
N$218
  Top 0.406: U$23.P$3 116.35,42.75 115.8,42.2 113.83,42.2 SV1.22
N$219
  Top 0.406: U$20.P$3 122.95,40.65 122.2,41.4 115.57,41.4 SV1.21
N$220
  Top 0.406: U$19.P$3 119.25,38.65 118.2,39.7 113.87,39.7 SV1.20
N$221
  Top 0.406: U$21.P$3 119.25,34.55 116.7,37.1 113.81,37.1 SV1.18
N$222  (via drill 0.4)
  Top 0.406: v105.1,80.7 102.76,80.7 U$50.P$3
  Bottom 0.406: SV1.49 114.87,76.47 113.7,75.3 110.7,75.3 110.6,75.2 110.6,68.3 108.8,66.5 103.7,66.5 101.9,68.3 101.9,74.8 100.1,76.7 100.1,77.7 100.7,78.2 104.6,78.2 105.1,78.7 v105.1,80.7
N$223
  Top 0.406: R62.2 122.6,47.54 U$25.P$1
N$224
  Top 0.406: U$22.P$3 122.75,36.45 121.8,37.4 119.2,37.4 118.1,38.5 115.21,38.5 SV1.19
N$225
  Top 0.406: SV1.31 113.79,54.9 111.9,54.9 111.3,54.3 111.3,53.3 109.8,51.8 109.8,47.7 109,46.9 106.4,46.9 105.64,47.66 U$32.P$3
N$226  (via drill 0.4)
  Top 0.406: U$31.P$3 100.85,49.75 v101.5,49.1
  Bottom 0.406: v101.5,49.1 105,49.1 107.3,51.4 112.21,51.4 SV1.30
N$227  (via drill 0.4)
  Top 0.406: U$28.P$3 104.55,51.95 v105.1,52.5
  Bottom 0.406: v105.1,52.5 111.8,52.5 111.9,52.4 113.75,52.4 SV1.29
N$228  (via drill 0.4)
  Top 0.406: U$27.P$3 101.75,54.05 102.6,53.2 104.3,53.2 104.6,53.5 105.7,53.5 106.4,52.8 v106.4,48.7
  Bottom 0.406: v106.4,48.7 112.37,48.7 SV1.28
N$229  (via drill 0.4)
  Top 0.406: U$29.P$3 99.75,58.25 v100.3,57.7 | v101.1,43.3 108.4,43.3 111.1,46 SV1.26
  Bottom 0.406: v100.3,57.7 100.3,44.1 v101.1,43.3
N$230
  Top 0.406: U$58.P$3 117.13,98.87 118.2,97.8 118.2,89.75 SV1.57
N$231
  Top 0.406: R70.2 96.68,44.81 U$33.P$1
N$232  (via drill 0.4)
  Top 0.406: U$30.P$3 105.85,56.05 107.6,54.3 v107.6,49.8
  Bottom 0.406: v107.6,49.8 113.81,49.8 SV1.27
N$233
  Top 0.406: IC5.17 131.69,57.41 R75.1
N$234
  Top 0.406: IC5.15 130.26,59.95 R73.1
N$235
  Top 0.406: R76.2 122.7,62.09 U$39.P$1
N$236
  Top 0.406: IC5.14 131.13,61.22 R76.1
N$237
  Top 0.406: R77.2 126.18,64.19 U$40.P$1
N$238
  Top 0.406: IC5.13 131.94,62.48 R77.1
N$239
  Top 0.406: IC5.12 132.85,63.76 R78.1
N$240
  Top 0.406: U$41.P$3 116.64,65.64 116.1,65.1 113.87,65.1 SV1.40
N$241
  Top 0.406: U$40.P$3 122.96,63.44 122.1,64.3 115.61,64.3 SV1.39
N$242
  Top 0.406: U$39.P$3 119.26,61.44 118.3,62.4 113.71,62.4 SV1.38
N$243
  Top 0.406: U$36.P$3 123.06,59.34 122.3,60.1 119.1,60.1 117.9,61.3 115.15,61.3 SV1.37
N$244
  Top 0.406: U$35.P$3 119.86,57.24 117.2,59.9 113.75,59.9 SV1.36
N$245
  Top 0.406: U$37.P$3 120.16,52.94 118.3,54.8 118.3,56.4 117.3,57.4 113.79,57.4 SV1.34
N$247
  Top 0.406: R78.2 122.56,66.39 U$41.P$1
N$248
  Top 0.406: U$38.P$3 122.86,55.14 122.2,55.8 120.1,55.8 117.2,58.7 SV1.35
N$249
  Top 0.406: IC6.17 130.79,74.47 R83.1
N$250
  Top 0.406: IC6.15 131.04,77 R81.1
N$251
  Top 0.406: R84.2 122.54,80.09 U$47.P$1
N$252
  Top 0.406: IC6.14 131.81,78.28 R84.1
N$253
  Top 0.406: R85.2 126.02,82.29 U$48.P$1
N$254
  Top 0.406: IC6.13 132.72,79.55 R85.1
N$255
  Top 0.406: IC6.12 133.53,80.81 R86.1
N$256
  Top 0.406: U$49.P$3 117.84,83.64 117.2,83 117.2,76.1 116.3,75.2 113.81,75.2 SV1.48
N$257
  Top 0.406: U$48.P$3 123.16,81.34 122.7,81.8 119.1,81.8 117.9,80.6 117.9,75.9 115.9,73.9 115.11,73.9 SV1.47
N$258
  Top 0.406: U$47.P$3 119.94,79.14 118.5,77.7 118.5,75.5 115.7,72.7 113.85,72.7 SV1.46
N$259
  Top 0.406: U$44.P$3 123.66,76.94 122.5,78.1 120,78.1 119.1,77.2 119.1,75.2 115.7,71.8 115.49,71.8 SV1.45
N$260
  Top 0.406: U$43.P$3 119.54,74.64 116.3,71.4 116.3,70.8 115.6,70.1 113.79,70.1 SV1.44
N$261
  Top 0.406: U$45.P$3 118.04,69.94 115.6,67.5 113.73,67.5 SV1.42
N$263
  Top 0.406: R86.2 122.7,84.39 U$49.P$1
N$264
  Top 0.406: U$46.P$3 123.36,72.44 122.4,73.4 119.3,73.4 116.9,71 116.9,70.4 115.8,69.3 115.53,69.3 SV1.43
N$265
  Top 0.406: R91.1 91.36,75.03 IC8.17
N$266
  Top 0.406: R89.1 91.33,72.48 IC8.15
N$267
  Top 0.406: R92.2 96.74,69.56 U$55.P$1
N$268
  Top 0.406: R92.1 90.47,71.22 IC8.14
N$269
  Top 0.406: R93.2 101.26,67.46 U$56.P$1
N$270
  Top 0.406: R93.1 89.66,69.94 IC8.13
N$271
  Top 0.406: R94.1 88.84,68.67 IC8.12
N$272
  Top 0.406: U$57.P$3 100.13,66.07 101.7,64.5 106.7,64.5 110.2,67.9 110.2,81.75 SV1.56
N$273
  Top 0.406: R98.2 97.26,95.96 U$61.P$1
N$274
  Top 0.406: IC9.18 91.52,94.44 R98.1
N$275  (via drill 0.4)
  Top 0.406: U$52.P$3 104.86,72.46 v105,72.5
  Bottom 0.406: SV1.53 113.83,82.8 111.6,82.8 106,77.2 106,74.3 105,73.3 v105,72.5
N$276  (via drill 0.4)
  Top 0.406: U$51.P$3 100.04,74.56 100.6,74 104,74 104.4,74.4 106.3,74.4 107.4,73.3 107.4,69.4 v107.3,69.3
  Bottom 0.406: v107.3,69.3 107.3,69.5 108.1,70.3 108.1,76 111.1,79 SV1.52
N$277
  Top 0.406: R99.2 100.88,93.86 U$62.P$1
N$278
  Bottom 0.406: JP1.3 3.32,56.32 4.5,57.5 10.1,57.5 12.6,55 27.4,55 29.1,56.7 29.1,58.7 29.9,59.5 U$68.2
N$279
  Top 0.406: R94.2 96.68,65.36 U$57.P$1
N$280  (via drill 0.4)
  Top 0.406: v104.3,76.9 102.89,76.9 U$54.P$3
  Bottom 0.406: SV1.51 115.01,79.01 113.8,77.8 111,77.8 109,75.8 109,68.9 108.2,68.1 104.4,68.1 103.4,69.1 103.4,69.9 104.1,70.6 104.1,72.7 103.8,73 103.8,74.6 104.3,75.1 v104.3,76.9
N$281
  Top 0.406: IC9.17 92.27,93.17 R99.1
N$282
  Top 0.406: IC9.15 91.86,90.62 R97.1
N$283
  Top 0.406: R100.2 94.45,87.55 arc-90 94.8,87.2 97.86,87.2 U$63.P$1
N$284
  Top 0.406: IC9.14 90.89,89.36 R100.1
N$285
  Top 0.406: R101.2 101.33,85.45 U$64.P$1
N$286
  Top 0.406: IC9.13 90.02,88.08 R101.1
N$287
  Top 0.406: IC9.12 89.14,86.81 R102.1
N$288
  Top 0.406: U$65.P$3 100.53,84.37 101.2,83.7 108.4,83.7 109.6,84.9 109.6,93.1 110.7,94.2 112.49,94.2 SV1.64
N$289
  Bottom 0.406: JP1.4 9.24,56.26 11.5,54 34.7,54 36.7,56 36.7,58.3 37.7,59.3 U$69.2
N$292  (via drill 0.4)
  Top 0.406: U$59.P$3 100.63,92.37 101.2,91.8 106.1,91.8 106.8,91.1 106.8,88.3 v107.4,87.7
  Bottom 0.406: v107.4,87.7 111.07,87.7 SV1.60
N$295
  Top 0.406: R102.2 97.55,83.35 U$65.P$1
N$296
  Top 0.406: U$62.P$3 104.77,94.57 106.6,96.4 115.2,96.4 116.3,95.3 116.3,90.39 SV1.59
VCC  (via drill 0.4)
  Top 0.406: U$65.P$2 100.33,82.77 v100.6,82.5 101.1,82 105.3,82 106.3,81 106.3,79.7 105.66,79.06 105.5,79.06 | v104.3,84.9 103.18,84.9 U$64.P$2 | U$63.P$2 100.53,86.87 v100.6,86.8 | U$60.P$2 103.67,88.97 v104.1,89.4 | U$59.P$2 100.37,90.77 v100.4,90.8 | U$62.P$2 104.03,92.97 v104.1,92.9 | U$61.P$2 100.33,95.07 v100.4,95 | U$58.P$2 103.77,97.27 v104,97.5 | 105.5,79.06 U$50.P$2 102.4,78.09 102.4,78 101.9,77.5 101.9,77.1 101.3,76.5 99.6,76.5 | U$54.P$2 104.67,75.07 105.3,75.7 105.3,78.86 105.5,79.06 | U$53.P$2 99.04,77.06 99.6,76.5 | 99.6,76.5 99.6,78.1 v99.4,78.3 | U$51.P$2 99.05,72.7 v99.9,72.7 100.5,73.3 105.5,73.3 106.1,72.7 106.1,71.5 105.46,70.86 U$52.P$2 | U$55.P$2 99.83,68.77 v99.9,68.7 | U$56.P$2 103.45,65.85 v103.1,65.5 | U$57.P$2 99.97,64.47 v100,64.5 | U$29.P$2 101.75,56.65 v102,56.9 103.1,56.9 104.3,58.1 104.3,58.72 U$26.P$2 | v101.8,52.4 98.8,52.4 U$27.P$2 | U$30.P$2 105.35,54.45 v105.5,54.6 | U$31.P$2 102.55,48.15 102.7,48.3 | 102.7,48.3 103,48.3 | 103,48.3 104.4,49.7 104.4,50.28 U$28.P$2 | v101.6,50.5 101.6,50.4 102.4,49.6 102.4,48.6 102.7,48.3 | 103,48.3 103,48.2 v102.8,48 | v101.7,45.7 101.7,45.4 102.1,45 104,45 104.4,45.4 104.4,45.95 U$32.P$2 | U$33.P$2 98.83,43.47 99.9,42.4 v102.4,42.4 | U$5.P$2 99.94,35.24 v100.1,35.4 | v99.7,30 99.7,30.05 U$3.P$2 | U$7.P$2 100.04,26.94 v100.1,27 | v100,22.6 99.96,22.64 U$9.P$2 98.83,21.8 | U$2.P$2 105.16,37.14 105.2,37.1 105.3,37.1 v105.4,37 | U$6.P$2 105.46,32.94 v105.7,32.7 | U$4.P$2 104.86,28.84 v105.2,28.5 | U$8.P$2 104.41,24.01 v103.9,23.5 | U$48.P$2 122.96,82.94 v122.9,83 | v120.5,86.7 120.5,85.29 U$49.P$2 | U$47.P$2 119.84,80.74 v119.3,80.2
  Top 0.406: U$44.P$2 123.46,78.54 v123.1,78.9 | U$43.P$2 120.57,76.87 v120.9,77.2 | U$46.P$2 123.36,74.04 v122.9,74.5 | U$45.P$2 120.53,72.03 120.9,72.4 v121.1,72.4 | U$42.P$2 123.14,70.34 v122.9,70.1 | U$41.P$2 119.34,67.24 v119,66.9 | U$40.P$2 122.84,65.04 v122.8,65 | U$39.P$2 119.36,63.04 v119.3,63.1 | U$36.P$2 122.86,60.94 v122.8,61 | U$35.P$2 119.66,58.84 v119.5,59 | U$38.P$2 122.94,56.74 v122.9,56.7 | U$37.P$2 119.96,54.54 v119.4,55.1 | U$34.P$2 122.74,52.54 v122.7,52.5 | U$25.P$2 120.29,49.39 v120.4,49.5 | U$24.P$2 122.55,46.35 v122.4,46.5 | U$23.P$2 119.25,44.35 v118.9,44 | U$20.P$2 122.45,42.25 v122.4,42.3 | U$19.P$2 119.05,40.25 v118.9,40.4 | U$22.P$2 122.65,38.05 v122.6,38.1 | U$21.P$2 119.15,36.15 v118.8,36.5 | U$18.P$2 122.45,33.95 v122.4,34 | U$17.P$2 119.95,32.45 v120,32.5 | U$16.P$2 122.75,29.25 v122.6,29.4 | U$12.P$2 122.75,25.05 v122.5,25.3 | U$11.P$2 119.77,23.23 v119.2,23.9 | U$14.P$2 122.75,20.95 v122.5,21.2 | U$13.P$2 119.73,18.97 v119,19.7 | U$10.P$2 122.25,16.85 v122.1,16.7 | 22.8,76.2 22.8,74.6 21.44,73.24 C7.2 21.38,72.91 C9.2 | 22.8,76.2 22.4,76.6 21.08,76.6 C8.2 20.4,77.28 v20.4,79.4 | IC10.20 14.18,78.17 14.7,78.7 | 14.7,78.7 14.7,84 v11.9,86.8 | v10,86.8 9.1,86.8 8.1,85.8 8.1,82.2 7.3,81.4 5.89,81.4 IC10.4 | 14.7,78.7 15.1,78.7 v16.4,80 | 47.56,78.96 IC14.5 36.14,78.96 34.8,80.3 34.11,80.3 C1.2 33.9,80.51 33.9,81.5 30.9,84.5 R1.1 30.54,84.4 29.6,84.4 28.8,85.2 | 47.56,78.96 47.85,79.25 | 47.85,79.25 48.2,79.6 48.1,79.7 IC14.38 48.1,92.1 47.76,92.44 R20.1 | 47.85,79.25 49.74,77.36 IC14.27 57.89,77.36 C3.1 58.44,71.65 R13.2 58.46,71.59 R12.2 58.46,69.36 57.4,68.3 57.4,62.6 56.4,61.6 56.4,57.5 57.4,56.5 57.4,39.4 v55.3,37.3
  Top 0.406: 47.56,78.96 47.3,78.7 IC14.17 47.3,69.7 46.5,68.9 46.5,64.3 48.19,62.62 IC11.PH 46.38,60.45 C22.2 | JP3.2 27.52,95.98 28.8,94.7 28.8,85.2 | 22.8,76.2 22.8,81.6 26.4,85.2 28.8,85.2 | IC1.4 50.51,24.39 51.5,23.4 | 51.5,23.4 52.8,22.1 55.63,22.1 IC1.18 60.29,21.99 | 51.5,23.4 50.89,22.79 IC1.6 47.15,22.8 45.2,22.8 44.46,23.54 C16.1 43.73,23.6 42.6,23.6 42.1,24.1 42.1,27.1 40.7,28.5 | IC12.1 C10.2 20.2,17.53 20.2,18.9 20.55,19.25 R15.1 26.12,26.12 | 60.29,21.99 C17.1 | 60.29,21.99 60.29,14.71 61.6,13.4 64.63,13.4 R18.A | R19.2 44.24,5.54 43.2,4.5 43.2,3.2 44.3,2.1 61.07,2.1 JP6.2 63.24,3.44 64.6,4.8 64.6,13.29 R18.A | 98.83,21.8 98.83,21.67 105.6,14.9 105.6,11.9 106.8,10.7 120.6,10.7 v122.1,12.2 122.6,11.7 132.7,11.7 134.69,13.69 134.69,16.71 | 26.12,26.12 28.7,28.7 40.5,28.7 40.7,28.5 | JP1.10 5.86,45.94 8,43.8 8,40.53 JP2.2 8.5,40.5 22.8,26.2 26.04,26.2 26.12,26.12 | IC9.20 84.28,96.97 83.8,96.5 83.8,84.35 C23.2 82.35,79.45 83.5,78.3 | IC8.20 84.03,78.83 83.5,78.3 | 83.5,78.3 83.3,78.1 83.3,66.35 C24.2 82.05,59.65 83.6,58.1 | IC4.20 83.77,58.27 83.6,58.1 | 83.6,58.1 82.5,57 82.5,44.45 C25.2 82.05,37.25 82.9,36.4 | IC7.20 83.19,36.69 82.9,36.4 | 82.9,36.4 82.4,35.9 82.4,22.85 C26.2 | C26.2 82.6,22.7 83.6,21.7 98.73,21.7 98.83,21.8 | C26.2 84,22.7 v84.5,23.2 | v82.6,13.4 64.71,13.4 R18.A | IC2.20 134.69,16.71 | 134.69,16.71 135.7,15.7 C27.2 137.2,17.25 137.2,32.4 | C28.2 137.2,32.6 | 137.2,32.6 137.17,32.6 IC3.20 134.72,35.08 137.2,32.6 | 137.2,32.6 137.2,32.4 | 137.2,32.4 137.4,32.6 137.4,46.7 138.85,48.15 C29.2 137.49,51 137.29,51.19 | 137.29,51.19 IC5.20 | 137.29,51.19 137.6,51.5 137.6,65.3 138.95,66.65 C30.2 137.45,68.2 IC6.20
  Top 0.406: v49.5,35.9 49.5,31.3 47.2,29 41.2,29 40.7,28.5 | U$15.P$2 119.85,27.25 v119.3,27.8
  Bottom 0.406: v100.6,82.5 101.9,82.5 v104.3,84.9 102.4,86.8 v100.6,86.8 103.2,89.4 103.4,89.4 | v104.1,89.4 103.4,89.4 | v100.4,90.8 102,90.8 | 102,90.8 103.4,89.4 | v104.1,92.9 103.75,92.55 | 103.75,92.55 102,90.8 | v100.4,95 100.9,95 | 100.9,95 101.3,95 103.75,92.55 | v104,97.5 103.4,97.5 100.9,95 | v99.4,78.3 99.4,73.2 v99.9,72.7 v99.9,68.7 v103.1,65.5 102.1,64.5 | v100,64.5 102.1,64.5 | 102,54.7 v102,56.9 102.1,57 102.1,64.5 | 102,54.7 102,52.6 | 102,52.6 v101.8,52.4 | v105.5,54.6 102.1,54.6 102,54.7 | 102,52.6 102,50.9 v101.6,50.5 | v102.8,48 102.8,46.8 v101.7,45.7 102.4,45 v102.4,42.4 105.4,39.4 v105.4,37 105.4,36.3 104.65,35.55 | 104.65,35.55 104.5,35.4 v100.1,35.4 100.1,30.4 v99.7,30 100.1,29.6 v100.1,27 100,26.9 v100,22.6 100.9,23.5 v103.9,23.5 | 104.65,35.55 105.7,34.5 v105.7,32.7 105.2,32.2 v105.2,28.5 | v120.5,86.7 122.9,84.3 v122.9,83 120.7,83 119.3,81.6 v119.3,80.2 120.6,78.9 | v123.1,78.9 120.6,78.9 | 120.6,78.9 120.9,78.6 v120.9,77.2 122.9,75.2 v122.9,74.5 121.1,72.7 v121.1,72.4 122.9,70.6 v122.9,70.1 121.4,68.6 119.4,68.6 119,68.2 v119,66.9 120.9,65 121,65 | v122.8,65 121,65 | 121,65 119.3,63.3 v119.3,63.1 120.65,61.75 | v122.8,61 121.4,61 120.65,61.75 | 120.65,61.75 119.5,60.6 v119.5,59 121,57.5 | v122.9,56.7 121.8,56.7 121,57.5 | 121,57.5 119.4,55.9 v119.4,55.1 122,52.5 | v122.7,52.5 122,52.5 | 122,52.5 120.4,50.9 v120.4,49.5 122.4,47.5 v122.4,46.5 119.9,44 v118.9,44 120.45,42.45 | v122.4,42.3 120.6,42.3 120.45,42.45 | 120.45,42.45 118.9,40.9 v118.9,40.4 120.55,38.75 | v122.6,38.1 121.2,38.1 120.55,38.75 | 120.55,38.75 118.8,37 v118.8,36.5 121.3,34 v122.4,34 120.9,32.5 v120,32.5 119.95,32.45 U$17.P$2 121.6,29.9
  Bottom 0.406: v122.6,29.4 122.1,29.4 121.6,29.9 | v119.3,27.8 119.5,27.8 | 119.5,27.8 121.6,29.9 | v119.2,23.9 121,23.9 121.15,23.95 | 121.15,23.95 v122.5,25.3 121.8,25.3 119.5,27.6 119.5,27.8 | 121.15,23.95 122.5,22.6 v122.5,21.2 121,19.7 | v119,19.7 121,19.7 | 121,19.7 122.1,18.6 v122.1,16.7 v122.1,12.2 | v11.9,86.8 v10,86.8 | v16.4,80 19.8,80 v20.4,79.4 | v84.5,23.2 84.5,15.3 v82.6,13.4 | v55.3,37.3 50.9,37.3 v49.5,35.9

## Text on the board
Top: ISP 1 | TOP | LED Cube | PC | LAYER | 12V | ISP 2 | www.xythobuz.org
Bottom: BOTTOM | LED Cube | www.xythobuz.org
